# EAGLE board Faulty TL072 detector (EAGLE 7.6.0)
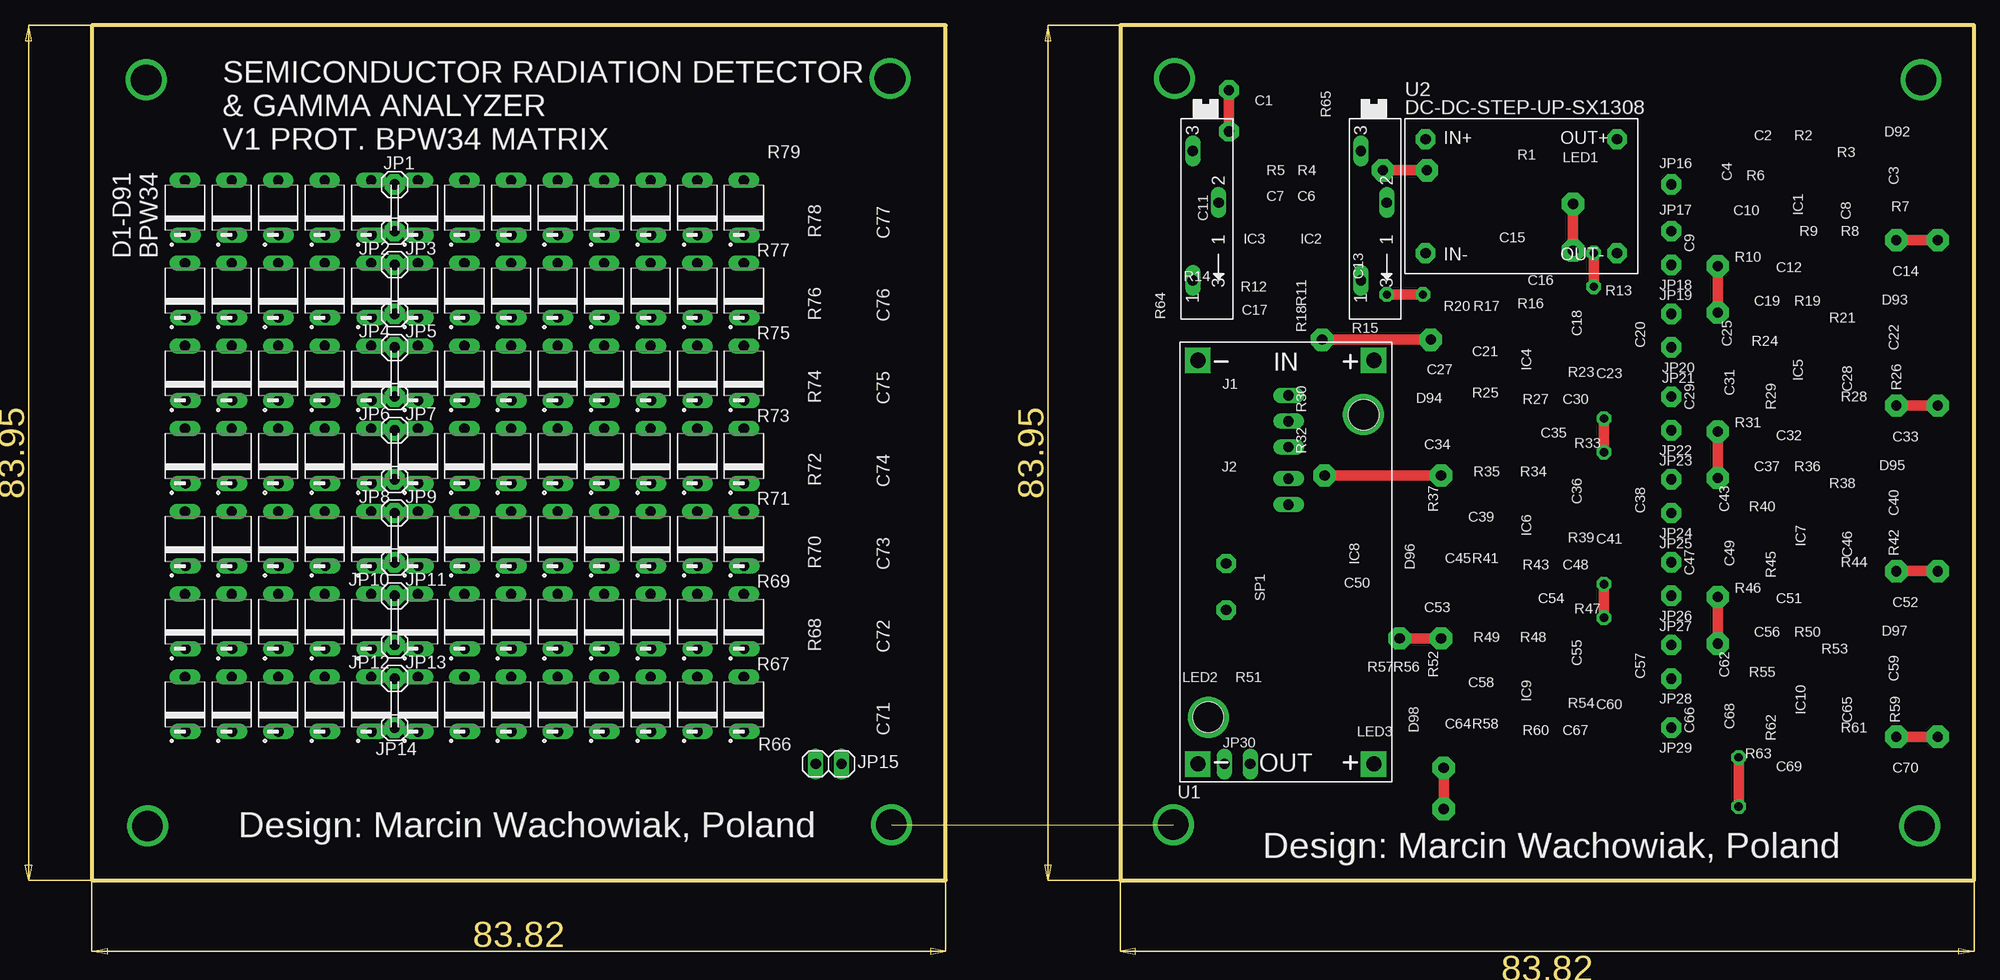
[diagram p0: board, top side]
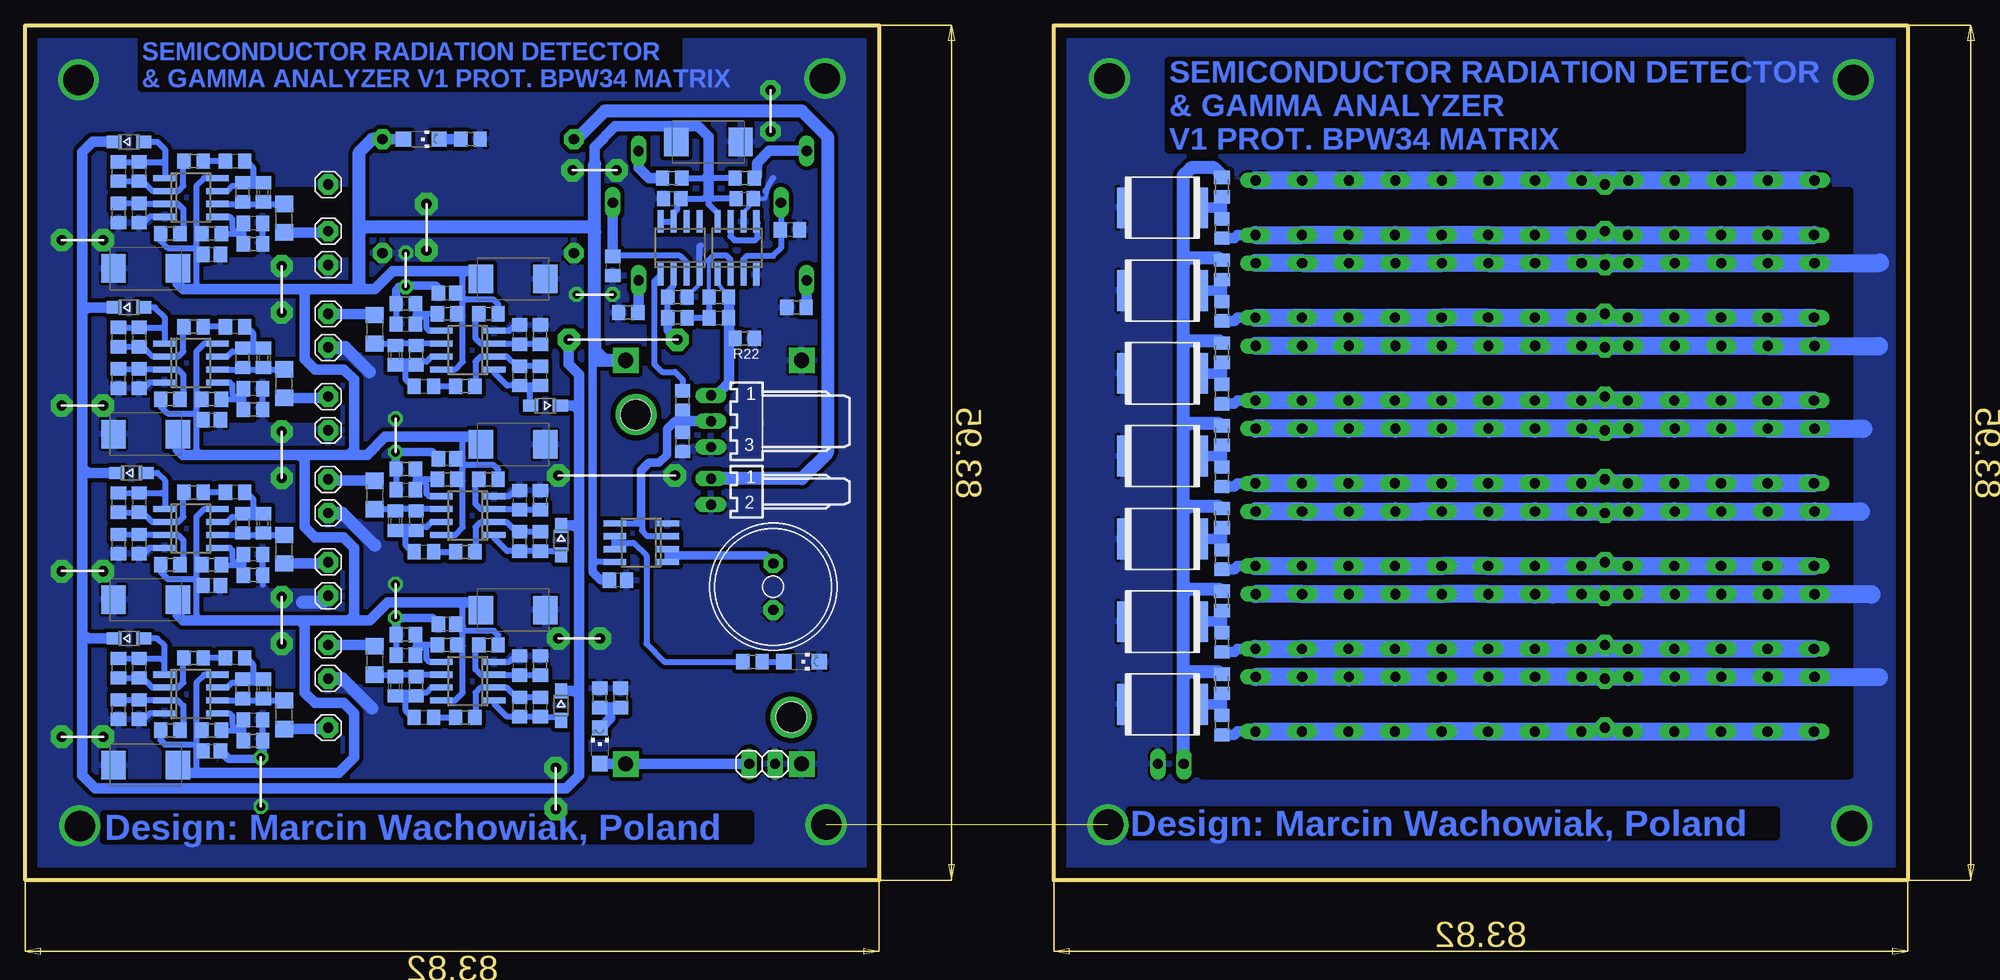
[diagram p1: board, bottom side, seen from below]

Size 191.31 x 91.23 mm. Coordinates in mm from the lower left corner, seen from the top.
Outline: 6.52,91.23 6.52,7.29 90.34,7.29 90.34,91.23 6.52,91.23
Outline: 191.31,91.23 107.49,91.23 107.49,7.29 191.31,7.29 191.31,91.23
Copper layers (1*16): Top 0.035mm / dielectric 1.5mm / Bottom 0.035mm
Design rules "default": minimum track width 10mil, minimum drill 24mil, track to track 8mil, track to pad 8mil, pad to pad 8mil, via to via 8mil, smd to smd 8mil, copper to edge 40mil, drill to drill 8mil, minimum pad ring 10mil, minimum via ring 8mil, stop-mask expansion 4mil, vias tented up to drill 0mil, thermal gap 10mil
bRestrict: area 159.6,68.9 to 166.9,75; area 160.8,36.4 to 167.2,40.2; area 160.8,20.6 to 167.2,24.4; area 160.8,19.3 to 167.2,20.6; area 160.8,52.6 to 167.2,56.7; area 155,59.5 to 162.9,64.6; area 155,43.2 to 162.9,48.3; area 155,27 to 162.9,32.1; area 12.2,17.6 to 72.4,75; area 72.4,22.7 to 75.7,75.7; area 72.4,17.6 to 75.7,22.7; area 167.2,18.7 to 172,20.6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

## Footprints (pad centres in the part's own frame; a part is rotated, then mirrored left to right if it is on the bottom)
SMC_D = smd 2.4 x 2.8: + -3.15,0; - 3.15,0
C0805 = smd 1.3 x 1.5: 1 -0.95,0; 2 0.95,0
C0603 = smd 1.1 x 1: 1 -0.85,0; 2 0.85,0
C0805' = smd 1.3 x 1.5: 1 -0.85,0; 2 0.85,0
C1206 = smd 1.6 x 1.8: 1 -1.4,0; 2 1.4,0
2824 = smd 1.2 x 4: 1 -3.85,0; 2 3.85,0
PHODET_BPW34 = drill 1 long: A 2.699,0.001; C -2.667,-0.033
SOD323-W = smd 1.5 x 1.2: A 1.45,0; C -1.45,0
SO08 = smd 0.6 x 2.2: 1 -1.905,-2.6; 2 -0.635,-2.6; 3 0.635,-2.6; 4 1.905,-2.6; 5 1.905,2.6; 6 0.635,2.6; 7 -0.635,2.6; 8 -1.905,2.6
7395-03 = drill 1.016 long: 1 2.54,0; 2 0,0; 3 -2.54,0
7395-02 = drill 1.016 long: 1 1.27,0; 2 -1.27,0
1X01 = drill 1.016 pad 2 octagon: 1 0,0
1X02 = drill 1.016 long: 1 -1.27,0; 2 1.27,0
CHIPLED_1206 = smd 1.5 x 1.5: A 0,-1.75; C 0,1.75
R0805 = smd 1.3 x 1.5: 1 -0.95,0; 2 0.95,0
SP19L = drill 1.016 long: A 5.715,-1.27; E -6.985,-1.27; S -1.905,1.27
M0805 = smd 1.3 x 1.6: 1 -0.95,0; 2 0.95,0
AL11P = drill 1.016 pad 1.905 octagon: + 2.286,0; - -2.286,0
DC-DC-STEP-DOWN-LM2596 = drill 1.5 pad 2.5 square: IN+ -19.812,8.636; IN- -19.812,-8.636; OUT+ 19.812,8.636; OUT- 19.812,-8.636 | hole 3: -14.478,7.62; 15.24,-7.62
DC-DC-STEP-UP-SX1308 = drill 1 pad 1.93 octagon: IN+ -9.398,5.588; IN- -9.398,-5.588; OUT+ 9.398,5.588; OUT- 9.398,-5.588

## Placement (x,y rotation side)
C1  100u/25V  [SMC_D]  124.25,79.8 0 bottom
C2  22n  [C0805]  170.73,77.9 180 bottom
C3  10p  [C0805]  182.16,76.88 270 bottom
C4  0,5pF  [C0603]  167.94,74.85 270 bottom
C5  0,5/1p  [C0805]  167.94,74.85 270 bottom
C6  100n  [C0805']  127.81,74.21 180 bottom
C7  100n  [C0805']  120.7,74.21 0 bottom
C8  100n  [C0805]  180.13,72.82 90 bottom
C9  100n/100V  [C1206]  165.91,72.31 90 bottom
C10  100n  [C0805]  168.96,71.8 180 bottom
C11  100n  [C0805]  116.25,71.17 180 bottom
C12  100n  [C0805']  173.02,68.75 0 bottom
C13  100n  [C0805]  133.65,67.61 270 bottom
C14  100u/25V  [SMC_D]  179.5,67.36 180 bottom
C15  100u/25V  [SMC_D]  143.43,66.34 0 bottom
C16  100n  [C0805']  149.91,64.94 180 bottom
C17  10p  [C0805]  123.24,62.53 0 bottom
C18  100n  [C0805]  153.97,61.89 0 bottom
C19  22n  [C0805]  170.73,61.64 180 bottom
C20  100n/100V  [C1206]  157.02,61.39 270 bottom
C21  100n  [C0805]  142.79,60.88 270 bottom
C22  10p  [C0805]  182.16,60.62 270 bottom
C23  0,5pF  [C0603]  154.99,58.85 90 bottom
C24  0,5/1p  [C0805]  154.99,58.85 90 bottom
C25  0,5/1p  [C0603]  167.94,58.59 270 bottom
C26  0,5/1p  [C0805]  167.94,58.59 270 bottom
C27  10p  [C0805]  140.76,56.81 90 bottom
C28  100n  [C0805]  180.13,56.56 90 bottom
C29  100n/100V  [C1206]  165.91,56.05 90 bottom
C30  22n  [C0805]  152.19,55.8 0 bottom
C31  100n  [C0805]  168.96,55.55 180 bottom
C32  100n  [C0805']  173.02,52.5 0 bottom
C33  100u/25V  [SMC_D]  179.5,51.1 180 bottom
C34  100u/25V  [SMC_D]  143.43,50.08 0 bottom
C35  100n  [C0805']  149.91,48.69 180 bottom
C36  100n  [C0805]  153.97,45.64 0 bottom
C37  22n  [C0805]  170.73,45.39 180 bottom
C38  100n/100V  [C1206]  157.02,45.13 270 bottom
C39  100n  [C0805]  142.79,44.62 270 bottom
C40  10p  [C0805]  182.16,44.37 270 bottom
C41  0,5pF  [C0603]  154.99,42.59 90 bottom
C42  0,5/1p  [C0805]  154.99,42.59 90 bottom
C43  0,5pF  [C0603]  167.94,42.34 270 bottom
C44  0,5/1p  [C0805]  167.94,42.34 270 bottom
C45  10p  [C0805]  140.76,40.56 90 bottom
C46  100n  [C0805]  180.13,40.31 90 bottom
C47  100n/100V  [C1206]  165.91,39.8 90 bottom
C48  22n  [C0805]  152.19,39.54 0 bottom
C49  100n  [C0805]  168.96,39.29 180 bottom
C50  100n  [C0805']  133.14,36.75 180 bottom
C51  100n  [C0805']  173.02,36.24 0 bottom
C52  100u/25V  [SMC_D]  179.5,34.84 180 bottom
C53  100u/25V  [SMC_D]  143.43,33.83 0 bottom
C54  100n  [C0805']  149.91,32.43 180 bottom
C55  100n  [C0805]  153.97,29.38 0 bottom
C56  22n  [C0805]  170.73,29.13 180 bottom
C57  100n/100V  [C1206]  157.02,28.88 270 bottom
C58  100n  [C0805]  142.79,28.37 270 bottom
C59  10p  [C0805]  182.16,28.11 270 bottom
C60  0,5pF  [C0603]  154.99,26.34 90 bottom
C61  0,5/1p  [C0805]  154.99,26.34 90 bottom
C62  0,5pF  [C0603]  167.94,26.08 270 bottom
C63  0,5/1p  [C0805]  167.94,26.08 270 bottom
C64  10p  [C0805]  140.76,24.3 90 bottom
C65  100n  [C0805]  180.13,24.05 90 bottom
C66  100n/100V  [C1206]  165.91,23.54 90 bottom
C67  22n  [C0805]  152.19,23.29 0 bottom
C68  100n  [C0805]  168.96,23.03 180 bottom
C69  100n  [C0805']  173.02,19.98 0 bottom
C70  100u/25V  [SMC_D]  179.5,18.59 180 bottom
C71  2,2uF/100V  [2824]  79.67,24.56 180 bottom
C72  2,2uF/100V  [2824]  79.67,32.69 180 bottom
C73  2,2uF/100V  [2824]  79.67,40.81 180 bottom
C74  2,2uF/100V  [2824]  79.67,48.94 180 bottom
C75  2,2uF/100V  [2824]  79.67,57.07 180 bottom
C76  2,2uF/100V  [2824]  79.67,65.2 180 bottom
C77  2,2uF/100V  [2824]  79.67,73.33 180 bottom
D1  BPW34  [PHODET_BPW34]  15.67,73.33 90 top
D2  BPW34  [PHODET_BPW34]  20.24,73.33 90 top
D3  BPW34  [PHODET_BPW34]  24.81,73.33 90 top
D4  BPW34  [PHODET_BPW34]  29.38,73.33 90 top
D5  BPW34  [PHODET_BPW34]  33.95,73.33 90 top
D6  BPW34  [PHODET_BPW34]  38.53,73.33 90 top
D7  BPW34  [PHODET_BPW34]  43.1,73.33 90 top
D8  BPW34  [PHODET_BPW34]  47.67,73.33 90 top
D9  BPW34  [PHODET_BPW34]  52.24,73.33 90 top
D10  BPW34  [PHODET_BPW34]  56.81,73.33 90 top
D11  BPW34  [PHODET_BPW34]  61.39,73.33 90 top
D12  BPW34  [PHODET_BPW34]  65.96,73.33 90 top
D13  BPW34  [PHODET_BPW34]  70.53,73.33 90 top
D14  BPW34  [PHODET_BPW34]  15.67,65.2 90 top
D15  BPW34  [PHODET_BPW34]  20.24,65.2 90 top
D16  BPW34  [PHODET_BPW34]  24.81,65.2 90 top
D17  BPW34  [PHODET_BPW34]  29.38,65.2 90 top
D18  BPW34  [PHODET_BPW34]  33.95,65.2 90 top
D19  BPW34  [PHODET_BPW34]  38.53,65.2 90 top
D20  BPW34  [PHODET_BPW34]  43.1,65.2 90 top
D21  BPW34  [PHODET_BPW34]  47.67,65.2 90 top
D22  BPW34  [PHODET_BPW34]  52.24,65.2 90 top
D23  BPW34  [PHODET_BPW34]  56.81,65.2 90 top
D24  BPW34  [PHODET_BPW34]  61.39,65.2 90 top
D25  BPW34  [PHODET_BPW34]  65.96,65.2 90 top
D26  BPW34  [PHODET_BPW34]  70.53,65.2 90 top
D27  BPW34  [PHODET_BPW34]  15.67,57.07 90 top
D28  BPW34  [PHODET_BPW34]  20.24,57.07 90 top
D29  BPW34  [PHODET_BPW34]  24.81,57.07 90 top
D30  BPW34  [PHODET_BPW34]  29.38,57.07 90 top
D31  BPW34  [PHODET_BPW34]  33.95,57.07 90 top
D32  BPW34  [PHODET_BPW34]  38.53,57.07 90 top
D33  BPW34  [PHODET_BPW34]  43.1,57.07 90 top
D34  BPW34  [PHODET_BPW34]  47.67,57.07 90 top
D35  BPW34  [PHODET_BPW34]  52.24,57.07 90 top
D36  BPW34  [PHODET_BPW34]  56.81,57.07 90 top
D37  BPW34  [PHODET_BPW34]  61.39,57.07 90 top
D38  BPW34  [PHODET_BPW34]  65.96,57.07 90 top
D39  BPW34  [PHODET_BPW34]  70.53,57.07 90 top
D40  BPW34  [PHODET_BPW34]  15.67,48.94 90 top
D41  BPW34  [PHODET_BPW34]  20.24,48.94 90 top
D42  BPW34  [PHODET_BPW34]  24.81,48.94 90 top
D43  BPW34  [PHODET_BPW34]  29.38,48.94 90 top
D44  BPW34  [PHODET_BPW34]  33.95,48.94 90 top
D45  BPW34  [PHODET_BPW34]  38.53,48.94 90 top
D46  BPW34  [PHODET_BPW34]  43.1,48.94 90 top
D47  BPW34  [PHODET_BPW34]  47.67,48.94 90 top
D48  BPW34  [PHODET_BPW34]  52.24,48.94 90 top
D49  BPW34  [PHODET_BPW34]  56.81,48.94 90 top
D50  BPW34  [PHODET_BPW34]  61.39,48.94 90 top
D51  BPW34  [PHODET_BPW34]  65.96,48.94 90 top
D52  BPW34  [PHODET_BPW34]  70.53,48.94 90 top
D53  BPW34  [PHODET_BPW34]  15.67,40.81 90 top
D54  BPW34  [PHODET_BPW34]  20.24,40.81 90 top
D55  BPW34  [PHODET_BPW34]  24.81,40.81 90 top
D56  BPW34  [PHODET_BPW34]  29.38,40.81 90 top
D57  BPW34  [PHODET_BPW34]  33.95,40.81 90 top
D58  BPW34  [PHODET_BPW34]  38.53,40.81 90 top
D59  BPW34  [PHODET_BPW34]  43.1,40.81 90 top
D60  BPW34  [PHODET_BPW34]  47.67,40.81 90 top
D61  BPW34  [PHODET_BPW34]  52.24,40.81 90 top
D62  BPW34  [PHODET_BPW34]  56.81,40.81 90 top
D63  BPW34  [PHODET_BPW34]  61.39,40.81 90 top
D64  BPW34  [PHODET_BPW34]  65.96,40.81 90 top
D65  BPW34  [PHODET_BPW34]  70.53,40.81 90 top
D66  BPW34  [PHODET_BPW34]  15.67,32.69 90 top
D67  BPW34  [PHODET_BPW34]  20.24,32.69 90 top
D68  BPW34  [PHODET_BPW34]  24.81,32.69 90 top
D69  BPW34  [PHODET_BPW34]  29.38,32.69 90 top
D70  BPW34  [PHODET_BPW34]  33.95,32.69 90 top
D71  BPW34  [PHODET_BPW34]  38.53,32.69 90 top
D72  BPW34  [PHODET_BPW34]  43.1,32.69 90 top
D73  BPW34  [PHODET_BPW34]  47.67,32.69 90 top
D74  BPW34  [PHODET_BPW34]  52.24,32.69 90 top
D75  BPW34  [PHODET_BPW34]  56.81,32.69 90 top
D76  BPW34  [PHODET_BPW34]  61.39,32.69 90 top
D77  BPW34  [PHODET_BPW34]  65.96,32.69 90 top
D78  BPW34  [PHODET_BPW34]  70.53,32.69 90 top
D79  BPW34  [PHODET_BPW34]  15.67,24.56 90 top
D80  BPW34  [PHODET_BPW34]  20.24,24.56 90 top
D81  BPW34  [PHODET_BPW34]  24.81,24.56 90 top
D82  BPW34  [PHODET_BPW34]  29.38,24.56 90 top
D83  BPW34  [PHODET_BPW34]  33.95,24.56 90 top
D84  BPW34  [PHODET_BPW34]  38.53,24.56 90 top
D85  BPW34  [PHODET_BPW34]  43.1,24.56 90 top
D86  BPW34  [PHODET_BPW34]  47.67,24.56 90 top
D87  BPW34  [PHODET_BPW34]  52.24,24.56 90 top
D88  BPW34  [PHODET_BPW34]  56.81,24.56 90 top
D89  BPW34  [PHODET_BPW34]  61.39,24.56 90 top
D90  BPW34  [PHODET_BPW34]  65.96,24.56 90 top
D91  BPW34  [PHODET_BPW34]  70.53,24.56 90 top
D92  1N4448  [SOD323-W]  181.15,79.8 0 bottom
D93  1N4448  [SOD323-W]  181.15,63.55 0 bottom
D94  1N4448  [SOD323-W]  140.25,53.89 180 bottom
D95  1N4448  [SOD323-W]  180.89,47.29 0 bottom
D96  1N4448  [SOD323-W]  138.73,40.69 270 bottom
D97  1N4448  [SOD323-W]  181.15,31.03 0 bottom
D98  1N4448  [SOD323-W]  138.73,24.43 270 bottom
IC1  TL072  [SO08]  175.05,74.34 270 bottom
IC2  LM311  [SO08]  127.05,69.39 0 bottom
IC3  LM358  [SO08]  121.46,69.39 0 bottom
IC4  TL072  [SO08]  147.87,59.36 90 bottom
IC5  TL072  [SO08]  175.05,58.09 270 bottom
IC6  TL072  [SO08]  147.87,43.1 90 bottom
IC7  TL072  [SO08]  175.05,41.83 270 bottom
IC8  LM358  [SO08]  130.86,40.43 90 bottom
IC9  TL072  [SO08]  147.87,26.84 90 bottom
IC10  TL072  [SO08]  175.05,25.57 270 bottom
J1  3pin  [7395-03]  124,52.37 90 bottom
J2  2pin  [7395-02]  124,45.45 90 bottom
JP1  [1X01]  36.24,75.61 0 top
JP2  [1X01]  36.24,71.04 0 top
JP3  [1X01]  36.24,67.74 0 top
JP4  [1X01]  36.24,62.91 0 top
JP5  [1X01]  36.24,59.61 0 top
JP6  [1X01]  36.24,54.78 0 top
JP7  [1X01]  36.24,51.48 0 top
JP8  [1X01]  36.24,46.66 0 top
JP9  [1X01]  36.24,43.35 0 top
JP10  [1X01]  36.24,38.53 0 top
JP11  [1X01]  36.24,35.23 0 top
JP12  [1X01]  36.24,30.4 0 top
JP13  [1X01]  36.24,27.1 0 top
JP14  [1X01]  36.24,22.27 0 top
JP15  GP  [1X02]  78.85,18.72 180 top
JP16  [1X01]  161.59,75.61 0 bottom
JP17  [1X01]  161.59,71.04 0 bottom
JP18  [1X01]  161.59,67.74 0 bottom
JP19  [1X01]  161.59,62.91 0 bottom
JP20  [1X01]  161.59,59.61 0 bottom
JP21  [1X01]  161.59,54.78 0 bottom
JP22  [1X01]  161.59,51.48 0 bottom
JP23  [1X01]  161.59,46.66 0 bottom
JP24  [1X01]  161.59,43.35 0 bottom
JP25  [1X01]  161.59,38.53 0 bottom
JP26  [1X01]  161.59,35.23 0 bottom
JP27  [1X01]  161.59,30.4 0 bottom
JP28  [1X01]  161.59,27.1 0 bottom
JP29  [1X01]  161.59,22.27 0 bottom
JP30  [1X02]  118.98,18.72 0 bottom
LED1  GREEN  [CHIPLED_1206]  152.45,80.06 270 bottom
LED2  RED  [CHIPLED_1206]  115.11,28.75 270 bottom
LED3  GREEN  [CHIPLED_1206]  134.92,20.49 0 bottom
R1  3k  [R0805]  147.62,80.06 0 bottom
R2  1k  [R0805]  174.8,77.9 0 bottom
R3  100k  [R0805]  180.13,76.88 270 bottom
R4  1k  [R0805]  127.81,76.25 180 bottom
R5  1k  [R0805]  120.7,76.25 180 bottom
R6  10M  [R0805]  169.97,74.85 270 bottom
R7  10k  [R0805]  182.16,72.82 270 bottom
R8  10k  [R0805]  177.08,70.78 0 bottom
R9  10k  [R0805]  173.02,70.78 0 bottom
R10  10k  [R0805]  168.96,69.77 0 bottom
R11  10k  [R0805]  127.3,64.56 0 bottom
R12  ***  [R0805]  123.24,64.56 0 bottom
R13  10k  [R0805]  153.97,63.93 180 bottom
R14  1k  [R0805]  115.62,63.55 0 bottom
R15  1k  [R0805]  132.13,63.04 180 bottom
R16  10k  [R0805]  149.91,62.91 180 bottom
R17  10k  [R0805]  145.84,62.91 180 bottom
R18  10k  [R0805]  127.3,62.53 0 bottom
R19  1k  [R0805]  174.8,61.64 0 bottom
R20  10k  [R0805]  140.76,60.88 90 bottom
R21  100k  [R0805]  180.13,60.62 270 bottom
R22  10k  [R0805]  120.7,60.5 180 bottom
R23  10M  [R0805]  152.95,58.85 90 bottom
R24  10M  [R0805]  169.97,58.59 270 bottom
R25  100k  [R0805]  142.79,56.81 90 bottom
R26  10k  [R0805]  182.16,56.56 270 bottom
R27  1k  [R0805]  148.13,55.8 180 bottom
R28  10k  [R0805]  177.08,54.53 0 bottom
R29  10k  [R0805]  173.02,54.53 0 bottom
R30  1200  [R0805]  126.79,54.4 270 bottom
R31  10k  [R0805]  168.96,53.51 0 bottom
R32  560  [R0805]  126.79,50.34 270 bottom
R33  10k  [R0805]  153.97,47.67 180 bottom
R34  10k  [R0805]  149.91,46.66 180 bottom
R35  10k  [R0805]  145.84,46.66 180 bottom
R36  1k  [R0805]  174.8,45.39 0 bottom
R37  10k  [R0805]  140.76,44.62 90 bottom
R38  100k  [R0805]  180.13,44.37 270 bottom
R39  10M  [R0805]  152.95,42.59 90 bottom
R40  10M  [R0805]  169.97,42.34 270 bottom
R41  100k  [R0805]  142.79,40.56 90 bottom
R42  10k  [R0805]  182.16,40.31 270 bottom
R43  1k  [R0805]  148.13,39.54 180 bottom
R44  10k  [R0805]  177.08,38.27 0 bottom
R45  10k  [R0805]  173.02,38.27 0 bottom
R46  10k  [R0805]  168.96,37.26 0 bottom
R47  10k  [R0805]  153.97,31.41 180 bottom
R48  10k  [R0805]  149.91,30.4 180 bottom
R49  10k  [R0805]  145.84,30.4 180 bottom
R50  1k  [R0805]  174.8,29.13 0 bottom
R51  470  [R0805]  119.93,28.75 180 bottom
R52  10k  [R0805]  140.76,28.37 90 bottom
R53  100k  [R0805]  180.13,28.11 270 bottom
R54  10M  [R0805]  152.95,26.34 90 bottom
R55  10M  [R0805]  169.97,26.08 270 bottom
R56  20k  [R0805]  134.92,25.19 90 bottom
R57  20k  [R0805]  132.89,25.19 90 bottom
R58  100k  [R0805]  142.79,24.3 90 bottom
R59  10k  [R0805]  182.16,24.05 270 bottom
R60  1k  [R0805]  148.13,23.29 180 bottom
R61  10k  [R0805]  177.08,22.02 0 bottom
R62  10k  [R0805]  173.02,22.02 0 bottom
R63  10k  [R0805]  168.96,21 0 bottom
R64  100-330 prec  [SP19L]  115.87,71.93 270 top
R65  100-330 prec  [SP19L]  132.38,71.93 270 top
R66  100M  [R0805]  73.83,22.52 270 bottom
R67  1M  [M0805]  73.83,26.59 270 bottom
R68  100M  [R0805]  73.83,30.65 270 bottom
R69  1M  [M0805]  73.83,34.72 270 bottom
R70  100M  [R0805]  73.83,38.78 270 bottom
R71  1M  [M0805]  73.83,42.84 270 bottom
R72  100M  [R0805]  73.83,46.91 270 bottom
R73  1M  [M0805]  73.83,50.97 270 bottom
R74  100M  [R0805]  73.83,55.04 270 bottom
R75  1M  [M0805]  73.83,59.1 270 bottom
R76  100M  [R0805]  73.83,63.17 270 bottom
R77  1M  [M0805]  73.83,67.23 270 bottom
R78  100M  [R0805]  73.83,71.29 270 bottom
R79  1M  [M0805]  73.83,75.36 270 bottom
SP1  BUZ  [AL11P]  117.9,36.11 90 bottom
U1  DC-DC-STEP-UP-LM2596  [DC-DC-STEP-DOWN-LM2596]  123.74,38.53 270 top
U2  DC-DC-STEP-UP-SX1308  [DC-DC-STEP-UP-SX1308]  146.86,74.47 0 top

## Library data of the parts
C1-C5 C8-C11 C13-C15 C17-C31 C33 C34 C36-C49 C52 C53 C55-C68 C70 R1-R63 R66-R79 = rcl
C6 C7 C12 C16 C32 C35 C50 C51 C54 C69 = resistor
C71-C77 = capacitor-wima
D1-D91 = BPW34; AVAILABILITY: Good; DESCRIPTION: 950 nm 100 ns %C2%B1 65%C2%B0 Wide Angle Half Sensitivity TO-5 Silicon PIN Photodiode; MF: Vishay; MP: BPW34; PACKAGE: SMD-2 Vishay; PRICE: 0.62 USD
D92-D98 = diode
IC1-IC10 = linear
J1 = con-molex; OC_FARNELL: unknown; OC_NEWARK: unknown
J2 = con-molex; OC_FARNELL: 9731601; OC_NEWARK: unknown
JP1-JP30 = pinhead
LED1-LED3 = led
R64 R65 = pot
SP1 = buzzer; OC_FARNELL: unknown; OC_NEWARK: unknown
U1 U2 = diy-modules

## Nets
+18V: C1.+ C6.1 C7.1 C12.1 C14.+ C15.+ C16.1 C32.1 C33.+ C34.+ C35.1 C50.2 C51.1 C52.+ C53.+ C54.1 C69.1 C70.+ IC1.8 IC2.7 IC2.8 IC3.8 IC4.8 IC5.8 IC6.8 IC7.8 IC8.8 IC9.8 IC10.8 LED1.A R4.1 R5.2 R8.1 R9.1 R16.1 R17.1 R28.1 R29.1 R34.1 R35.1 R44.1 R45.1 R48.1 R49.1 R61.1 R62.1 U1.IN+ U2.OUT+
+24V: JP30.1 LED3.A U1.OUT+
+60: JP15.2 R67.1 R69.1 R71.1 R73.1 R75.1 R77.1 R79.1
A-OUT: C17.2 IC3.1 J1.1 R12.2 R22.2
D-OUT+5V: IC8.3 IC8.5 J1.2 R30.2 R32.1
GND: C1.- C6.2 C7.2 C8.1 C10.1 C11.1 C12.2 C13.2 C14.- C15.- C16.2 C18.1 C21.1 C28.1 C31.1 C32.2 C33.- C34.- C35.2 C36.1 C39.1 C46.1 C49.1 C50.1 C51.2 C52.- C53.- C54.2 C55.1 C58.1 C65.1 C68.1 C69.2 C70.- C71.2 C72.2 C73.2 C74.2 C75.2 C76.2 C77.2 D1.A D2.A D3.A D4.A D5.A D6.A D7.A D8.A D9.A D10.A D11.A D12.A D13.A D14.A D15.A D16.A D17.A D18.A D19.A D20.A D21.A D22.A D23.A D24.A D25.A D26.A D27.A D28.A D29.A D30.A D31.A D32.A D33.A D34.A D35.A D36.A D37.A D38.A D39.A D40.A D41.A D42.A D43.A D44.A D45.A D46.A D47.A D48.A D49.A D50.A D51.A D52.A D53.A D54.A D55.A D56.A D57.A D58.A D59.A D60.A D61.A D62.A D63.A D64.A D65.A D66.A D67.A D68.A D69.A D70.A D71.A D72.A D73.A D74.A D75.A D76.A D77.A D78.A D79.A D80.A D81.A D82.A D83.A D84.A D85.A D86.A D87.A D88.A D89.A D90.A D91.A IC1.4 IC2.4 IC3.4 IC3.6 IC4.4 IC5.4 IC6.4 IC7.4 IC8.4 IC9.4 IC10.4 J1.3 J2.2 JP1.1 JP3.1 JP5.1 JP7.1 JP9.1 JP11.1 JP13.1 JP15.1 JP16.1 JP18.1 JP20.1 JP22.1 JP24.1 JP26.1 JP28.1 JP30.2 LED2.C R1.2 R7.2 R10.2 R11.2 R13.2 R14.1 R15.2 R20.2 R22.1 R26.2 R31.2 R32.2 R33.2 R37.2 R42.2 R46.2 R47.2 R52.2 R56.2 R57.2 R59.2 R63.2 SP1.- U1.IN- U1.OUT- U2.IN- U2.OUT-
N$1: C10.2 IC1.5 R9.2 R10.1
N$3: C2.1 C4.1 C5.1 IC1.7 R6.1
N$4: J2.1 U2.IN+
N$5: C77.1 R78.1 R79.2
N$6: C8.2 IC1.3 R7.1 R8.2
N$7: C2.2 R2.2
N$8: C4.2 C5.2 C9.2 IC1.6 R6.2
N$9: C3.2 IC1.2 R2.1 R3.2
N$10: C3.1 D92.A IC1.1 R3.1
N$12: D92.C D93.C D94.C D95.C D96.C D97.C D98.C IC2.2 R11.1 R18.1
N$13: C76.1 R76.1 R77.2
N$14: C75.1 R74.1 R75.2
N$15: C74.1 R72.1 R73.2
N$16: C73.1 R70.1 R71.2
N$17: C72.1 R68.1 R69.2
N$18: C71.1 R66.1 R67.2
N$23: IC2.1 R30.1
N$24: C17.1 IC3.2 R12.1 R18.2
N$25: C13.1 IC2.3 R65.S
N$26: R4.2 R65.E
N$27: R15.1 R65.A
N$28: C25.2 C26.2 C29.2 IC5.6 R24.2
N$29: R5.1 R64.E
N$30: R14.2 R64.A
N$31: C11.2 IC3.3 R64.S
N$32: LED1.C R1.1
N$33: C31.2 IC5.5 R29.2 R31.1
N$34: LED3.C R56.1 R57.1
N$35: C19.1 C25.1 C26.1 IC5.7 R24.1
N$36: C19.2 R19.2
N$37: C22.2 IC5.2 R19.1 R21.2
N$38: C22.1 D93.A IC5.1 R21.1
N$39: C28.2 IC5.3 R26.1 R28.2
N$40: C38.2 C41.2 C42.2 IC6.6 R39.2
N$41: C36.2 IC6.5 R33.1 R34.2
N$42: C43.2 C44.2 C47.2 IC7.6 R40.2
N$43: C49.2 IC7.5 R45.2 R46.1
N$44: C37.1 C43.1 C44.1 IC7.7 R40.1
N$45: C37.2 R36.2
N$46: C40.2 IC7.2 R36.1 R38.2
N$47: C40.1 D95.A IC7.1 R38.1
N$48: C46.2 IC7.3 R42.1 R44.2
N$49: C41.1 C42.1 C48.1 IC6.7 R39.1
N$50: C48.2 R43.2
N$51: C62.2 C63.2 C66.2 IC10.6 R55.2
N$52: C68.2 IC10.5 R62.2 R63.1
N$53: C56.1 C62.1 C63.1 IC10.7 R55.1
N$54: C56.2 R50.2
N$55: C59.2 IC10.2 R50.1 R53.2
N$56: C59.1 D97.A IC10.1 R53.1
N$57: C65.2 IC10.3 R59.1 R61.2
N$58: C45.2 IC6.2 R41.2 R43.1
N$59: C45.1 D96.A IC6.1 R41.1
N$60: C20.2 C23.2 C24.2 IC4.6 R23.2
N$61: C18.2 IC4.5 R13.1 R16.2
N$62: C23.1 C24.1 C30.1 IC4.7 R23.1
N$63: C30.2 R27.2
N$64: C27.2 IC4.2 R25.2 R27.1
N$65: C27.1 D94.A IC4.1 R25.1
N$66: C21.2 IC4.3 R17.2 R20.1
N$67: C39.2 IC6.3 R35.2 R37.1
N$69: C57.2 C60.2 C61.2 IC9.6 R54.2
N$70: C55.2 IC9.5 R47.1 R48.2
N$71: C60.1 C61.1 C67.1 IC9.7 R54.1
N$72: C67.2 R60.2
N$73: C64.2 IC9.2 R58.2 R60.1
N$74: C64.1 D98.A IC9.1 R58.1
N$75: C58.2 IC9.3 R49.2 R52.1
N$78: IC8.1 IC8.2 SP1.+
N$79: IC8.6 IC8.7 R51.2
OUT1: D27.C D28.C D29.C D30.C D31.C D32.C D33.C D34.C D35.C D36.C D37.C D38.C D39.C JP6.1 R74.2
OUT3: D79.C D80.C D81.C D82.C D83.C D84.C D85.C D86.C D87.C D88.C D89.C D90.C D91.C JP14.1 R66.2
OUT4: D1.C D2.C D3.C D4.C D5.C D6.C D7.C D8.C D9.C D10.C D11.C D12.C D13.C JP2.1 R78.2
OUT5: D14.C D15.C D16.C D17.C D18.C D19.C D20.C D21.C D22.C D23.C D24.C D25.C D26.C JP4.1 R76.2
OUT9: D40.C D41.C D42.C D43.C D44.C D45.C D46.C D47.C D48.C D49.C D50.C D51.C D52.C JP8.1 R72.2
OUT10: C9.1 JP17.1
OUT12: C20.1 JP19.1
OUT13: C66.1 JP29.1
OUT14: C29.1 JP21.1
OUT15: C38.1 JP23.1
OUT16: C47.1 JP25.1
OUT17: C57.1 JP27.1
OUT21: D53.C D54.C D55.C D56.C D57.C D58.C D59.C D60.C D61.C D62.C D63.C D64.C D65.C JP10.1 R70.2
OUT22: D66.C D67.C D68.C D69.C D70.C D71.C D72.C D73.C D74.C D75.C D76.C D77.C D78.C JP12.1 R68.2
S$1: IC3.5 IC3.7
S$2: LED2.A R51.1

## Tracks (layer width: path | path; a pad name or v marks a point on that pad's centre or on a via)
+18V
  Bottom 0.61: IC4.8 149.14,57.45 148.38,58.21 148.38,62.78 | R16.1 148.51,62.91 148.38,62.78 | IC10.8 173.78,27.48 174.54,26.72 174.54,22.14 | C69.1 174,19.86 174.54,19.86 | R62.1 174.42,22.02 174.54,22.14 | IC7.8 173.78,43.73 174.54,42.97 174.54,38.4 | R45.1 174.42,38.27 174.54,38.4 | IC5.8 173.78,59.99 174.54,59.23 174.54,54.66 | C32.1 174,52.37 174.29,52.37 174.54,52.62 | R29.1 174.42,54.53 174.54,54.66 | IC1.8 173.78,76.25 174.54,75.48 174.54,70.91 | 174,68.63 C12.1 174.25,69.13 174.54,69.13 | R9.1 174.42,70.78 174.54,70.91 | 126.86,74.57 C6.1 | 126.86,79 C1.+ | IC6.8 149.14,41.19 148.38,41.96 148.38,46.53 | 148.38,46.53 148.38,48.05 | R34.1 148.51,46.66 148.38,46.53 | IC9.8 149.14,24.94 148.38,25.7 148.38,30.27 | 148.38,30.27 148.38,31.8 | R48.1 148.51,30.4 148.38,30.27 | 148.38,62.78 148.38,64.31 | 148.38,64.31 148.38,64.56 | 148.38,64.56 148.38,65.07 | C16.1 148.51,64.94 148.38,65.07 | 174.54,70.91 174.54,69.13 | 174.54,69.13 174.54,65.83 | 174.54,65.83 174.54,65.32 | R8.1 178.03,70.08 177.34,69.39 174.8,69.39 174.54,69.13 | R17.1 144.89,63.87 145.33,64.31 148.13,64.31 | 148.13,64.31 148.38,64.31 | 148.13,64.31 148.38,64.56 | 148.38,48.05 148.38,48.31 | 148.38,48.31 148.38,48.81 | 148.38,48.81 148.38,50.34 148.89,50.85 | 174.54,54.66 174.54,52.88 | 174.54,52.88 174.54,52.62 | 174.54,52.62 174.54,49.58 | R28.1 178.03,53.83 177.34,53.13 174.8,53.13 174.54,52.88 | R35.1 144.89,47.61 145.33,48.05 148.13,48.05 | 148.13,48.05 148.38,48.05 | 148.13,48.05 148.38,48.31 | C35.1 148.51,48.69 148.38,48.81 | 148.38,31.8 148.38,32.05 | 174.54,38.4 174.54,36.62 | 174.54,36.62 174.54,36.37 | 174.54,36.37 174.54,33.32 | 174.54,33.32 174.54,32.81
  Bottom 0.61: R44.1 178.03,37.57 177.34,36.88 174.8,36.88 174.54,36.62 | R49.1 144.89,31.35 145.33,31.8 148.13,31.8 | 148.13,31.8 148.38,31.8 | 148.13,31.8 148.38,32.05 | C51.1 174.42,36.24 174.54,36.37 | 148.38,32.05 148.38,32.3 | C54.1 148.51,32.43 148.38,32.3 | 148.38,32.3 148.38,34.08 148.89,34.59 | 174.54,33.32 174.29,33.07 174.29,32.81 | 174.54,49.07 174.54,49.58 | 174.54,49.58 173.78,49.07 | 174.54,65.83 174.04,65.32 | 148.38,65.07 148.38,66.59 148.89,67.1 | 174.54,22.14 174.54,20.37 | 174.54,20.37 174.54,19.86 | 174.54,19.86 174.54,18.33 174.04,17.83 | 177.08,18.08 176.85,18.08 C70.+ | R61.1 178.03,21.06 177.59,20.62 174.8,20.62 174.54,20.37 | IC2.8 IC2.7 127.68,72.82 127.3,73.2 127.3,73.87 C6.1 | R5.2 123.74,76.25 124.25,76.75 124.76,76.25 R4.1 | C6.1 124.76,74.21 | 124.76,74.21 124.51,74.47 | IC3.8 123.36,72.82 124.25,73.71 124.25,74.47 | 124.51,74.21 124.51,74.47 | 124.51,74.47 124.25,74.72 123.74,74.21 | C7.1 124.76,74.21 | 135.62,59.86 135.43,60.24 | IC8.8 135.24,38.53 135.62,38.91
  Bottom 0.813: 156.51,80.31 U2.OUT+ | 135.62,59.86 135.62,38.91 135.62,37.57 134.79,36.75 C50.2
  Bottom 1.016: C14.+ 176.35,65.86 175.81,65.32 174.54,65.32 174.04,65.32 164.38,65.32 | C33.+ 176.35,49.6 175.81,49.07 174.54,49.07 173.78,49.07 163.62,49.07 | C52.+ 176.35,33.34 175.81,32.81 174.54,32.81 174.29,32.81 164.38,32.81 | 164.38,32.81 159.56,32.81 | 159.56,32.81 159.3,32.81 | 159.56,49.07 159.05,49.58 159.05,56.43 160.07,57.45 162.86,57.45 163.88,58.47 163.88,65.07 164.38,65.32 | 159.43,32.94 159.05,33.32 159.05,39.92 160.07,40.94 162.86,40.94 163.88,41.96 163.88,48.56 164,48.69 | 159.43,32.94 159.56,32.81 | 164,48.69 164.38,49.07 | 159.56,49.07 163.62,49.07 | 163.62,49.07 164,48.69 | 159.3,32.81 159.43,32.94 | 176.09,18.33 C70.+ | 164.38,32.81 163.88,32.3 163.88,25.7 162.86,24.68 160.07,24.68 159.05,23.67 159.05,19.35 160.57,17.83 174.04,17.83 176.07,17.83 | 164.38,65.32 159.05,65.32 | 159.05,65.32 158.54,65.32 | 158.54,65.32 157.02,65.32 155.24,67.1 148.89,67.1 147.34,67.1 C15.+ | C1.+ 127.05,80.16 127.05,81.07 127.3,81.33 | 158.54,66.34 158.54,65.83 | 158.54,65.83 158.54,65.32 | 158.54,65.83 159.05,65.32 | LED1.A U2.OUT+ | 124.25,74.47 124.25,74.72 124.25,76.75 124.25,80.31 125.27,81.33 127.3,81.33 | 159.3,32.81 157.53,32.81 155.75,34.59 148.89,34.59 147.34,34.59 C53.+ | 159.56,49.07 157.78,49.07 156,50.85 148.89,50.85 147.34,50.85 C34.+ | 127.3,81.33 133.4,81.33 135.43,79.29 135.43,77.14
  Bottom 1.27: U2.OUT+ 157.27,80.06 158.54,78.79 158.54,70.91 | 158.54,65.83 158.54,70.91 | U1.IN+ 134.41,58.34 | 134.41,58.34 135.05,58.34 | 135.43,70.91 135.43,60.24 135.43,59.36 134.41,58.34 | 158.54,70.91 158.03,71.42 135.94,71.42 135.43,70.91 | 176.09,18.33 176.09,17.85 176.07,17.83 | 135.43,70.91 135.43,77.14 135.43,77.64
+24V
  Bottom 1.016: 134.76,18.72 LED3.A 134.89,18.72 U1.OUT+ JP30.1
+60
  Bottom 1.016: R69.1 73.83,35.76
  Bottom 1.27: R79.1 73.83,76.39 arc-45 73.91,76.57 74.59,77.26 76.78,77.26 arc-45 76.95,77.19 77.64,76.5 77.64,67.86 | 77.64,67.86 77.64,59.74 | 77.64,59.74 77.64,51.61 | 77.64,51.61 77.64,43.48 | 77.64,43.48 77.64,35.35 | 77.64,35.35 77.64,27.22 | 77.64,27.22 77.64,18.72 JP15.2 | R67.1 arc45 73.94,27.58 74.09,27.73 77.03,27.73 arc-45 77.21,27.66 77.64,27.22 | 73.83,35.76 73.88,35.76 arc45 74.06,35.83 74.09,35.86 77.03,35.86 arc-45 77.21,35.79 77.64,35.35 | R71.1 arc45 73.94,43.84 74.09,43.99 77.03,43.99 arc-45 77.21,43.91 77.64,43.48 | R73.1 arc45 73.94,51.97 74.09,52.12 77.03,52.12 arc-45 77.21,52.04 77.64,51.61 | R75.1 arc45 73.94,60.09 74.09,60.24 77.03,60.24 arc-45 77.21,60.17 77.64,59.74 | R77.1 arc45 73.94,68.22 74.09,68.37 77.03,68.37 arc-45 77.21,68.3 77.64,67.86
A-OUT
  Bottom 0.406: 123.24,65.83 IC3.1 | C17.2 R22.2
  Bottom 0.457: R12.2 123.24,65.83
  Bottom 0.61: R12.2 C17.2
  Bottom 1.016: R22.2 122.22,60.5 | 122.22,60.5 122.22,64.56 | 122.22,60.5 122.22,56.18 123.49,54.91 J1.1
D-OUT+5V
  Bottom 0.61: 130.79,42.46 130.79,42.91 130.86,42.97 131.49,42.34 | 130.79,42.46 130.79,41.64 130.22,41.07 IC8.3 | IC8.5 130.92,42.34 130.79,42.46
  Bottom 0.813: 124.25,52.37 J1.2 | 130.86,42.97 130.86,47.54 130.09,48.31 129.08,48.31 128.32,49.07 128.32,51.61 127.55,52.37 126.79,52.37
  Bottom 1.016: J1.2 126.54,52.37 126.79,52.62 R30.2 126.79,52.37 R32.1
GND  (via drill 0.8 pad 1.42, 1 pad 1.93, 1 pad 2.18, 3 pad 4)  (1 unrouted)
  Top 1.016: v187.75,70.15 v183.69,70.15 | v187.75,53.89 v183.69,53.89 | v187.75,37.64 v183.69,37.64 | v187.75,21.38 v183.69,21.38 | v166.16,63.04 v166.16,67.61 | v166.16,46.78 v166.16,51.35 | v166.16,30.53 v166.16,35.1 | v138.98,31.03 v134.92,31.03 | v154.99,33.07 v154.99,36.37 | v154.99,49.32 v154.99,52.62 | v153.97,65.58 v153.97,68.88 | v168.19,14.52 v168.19,19.35 | v139.24,14.27 v139.24,18.33 | v151.94,69.13 v151.94,73.71 | v138.98,47.04 v127.55,47.04 | v133.65,64.82 v137.21,64.82 | v133.27,77.01 v137.59,77.01 | v118.16,84.88 v118.16,80.82
  Bottom 0.406: 120.82,72.75 120.82,72.88 120.25,73.45 120.25,73.81 119.93,74.21 C7.2 118.66,74.21 118.26,75.65 | R11.2 126.35,64.62 125.14,65.83 IC2.4
  Bottom 0.61: R47.2 C55.1 | 151.14,32.81 C54.2 | IC9.4 143.81,28.75 143.3,29.26 142.85,29.26 C58.1 | C36.1 R33.2 154.92,48.63 | 151.14,49.07 C35.2 | IC6.4 143.81,45 143.3,45.51 142.85,45.51 C39.1 | R10.2 C10.1 | IC1.4 179.12,72.44 179.62,71.93 180.07,71.93 C8.1 | R31.2 C31.1 | IC5.4 179.12,56.18 179.62,55.67 180.07,55.67 C28.1 | C49.1 R46.2 168.01,36.3 | 171.79,35.86 C51.2 | IC7.4 179.12,39.92 179.62,39.42 180.07,39.42 C46.1 | R63.2 C68.1 | 171.79,19.6 C69.2 | IC10.4 179.12,23.67 179.62,23.16 180.07,23.16 C65.1 | R13.2 C18.1 | IC4.4 143.81,61.26 143.3,61.77 142.85,61.77 C21.1 | IC3.6 120.82,72.75 | IC2.4 125.14,69.52 125.01,69.64 | 118.66,74.98 118.26,75.65 117.9,76.25
  Bottom 0.813: 171.79,19.6 171.75,19.6 171.37,19.22 168.32,19.22 v168.19,19.35 168.01,19.54 R63.2 | C16.2 150.76,65.41 151.05,65.7 153.84,65.7 v153.97,65.58 154.6,65.58 154.92,65.26 R13.2 | 151.14,49.07 151.39,49.32 v154.99,49.32 154.99,47.74 R33.2 | C54.2 151.39,33.07 v154.99,33.07 154.92,33 R47.2
  Bottom 1.27: 161.59,35.1 162.1,34.59 164.13,34.59 | 157.53,57.2 159.94,59.61 JP20.1 | 157.02,40.18 160.19,43.35 JP24.1 | JP28.1 160.19,27.1 157.27,24.18
  Bottom 1.778: 36.24,27.26 D83.A D82.A D81.A D80.A D79.A 9.39,27.26 arc45 9.32,27.22 | 36.24,27.26 D84.A D85.A D86.A D87.A D88.A D89.A D90.A D91.A | D72.A D73.A D74.A D75.A D76.A D77.A D78.A | D72.A D71.A 35.99,35.38 | 35.99,35.38 D70.A D69.A D68.A D67.A D66.A 10.16,35.38 arc45 10.08,35.35 | D72.A 41.35,35.38 41.32,35.35 43.1,35.35 | 54.24,43.51 D62.A D63.A D64.A D65.A | 35.99,43.51 D58.A D59.A D60.A D61.A 54.24,43.51 | 35.99,43.51 D57.A D56.A D55.A D54.A D53.A 11.17,43.51 arc45 11.09,43.48 | 54.24,43.51 54.28,43.48 | D44.A D43.A D42.A D41.A D40.A 10.92,51.64 arc45 10.84,51.61 | D44.A 37.8,51.64 | 37.8,51.64 D45.A D46.A D47.A D48.A D49.A D50.A D51.A D52.A | 37.8,51.64 37.76,51.61 36.24,51.61 | 36.24,51.61 33.99,51.61 D44.A | 36.24,59.77 D31.A D30.A D29.A D28.A D27.A 9.39,59.77 arc45 9.32,59.74 | 36.24,59.77 D32.A D33.A D34.A D35.A D36.A D37.A D38.A D39.A | 35.99,67.9 D19.A D20.A D21.A D22.A D23.A D24.A D25.A D26.A | 35.99,67.9 D18.A D17.A D16.A D15.A D14.A 9.39,67.9 arc-45 9.21,67.97 | D13.A D12.A D11.A D10.A D9.A D8.A D7.A D6.A D5.A D4.A D3.A D2.A D1.A | JP11.1 arc-45 36.08,35.29 35.99,35.38 | JP13.1 36.24,27.26 | JP9.1 arc-45 36.08,43.42 35.99,43.51 | JP7.1 36.24,51.61 | JP3.1 arc-45 36.08,67.8 35.99,67.9 | JP5.1 36.24,59.77
  other vias: 186.1,85.9 112.82,86.03 185.97,12.62 112.69,12.75 11.86,85.9 11.98,12.62 85.01,12.75 84.88,86.03
  pour Bottom (isolate 0.406): 6.27,91.11 90.34,91.11 90.34,7.29 6.27,7.29
  pour Bottom (isolate 0.406): 191.31,91.11 107.23,91.11 107.49,7.29 191.31,7.29
N$1
  Bottom 0.61: R10.1 169.91,70.91 | 169.91,70.91 C10.2 | R9.2 170.48,70.78 | 170.48,70.78 170.03,70.78 169.91,70.91 | IC1.5 171.24,72.44 170.99,72.18 170.99,71.29 170.48,70.78
N$3
  Bottom 0.254: C5.1 C4.1
  Bottom 0.61: IC1.7 171.5,74.98 170.99,75.48 169.72,75.48 | 169.72,75.48 168.96,75.48 | 168.96,75.48 168.16,75.48 C4.1 | R6.1 169.97,75.74 169.72,75.48 | C2.1 169.59,77.9 168.96,77.26 168.96,75.48
N$4
  Bottom 1.27: U2.IN+ 137.21,80.06 134.41,82.85 115.11,82.85 112.57,80.31 112.57,49.26 115.11,46.72 J2.1
N$5
  Bottom 1.016: R79.2 73.83,73.45 | 73.83,73.45 R78.1 | C77.1 73.96,73.33 arc-90 73.83,73.45
N$6
  Bottom 0.61: R7.1 C8.2 180.07,73.71 IC1.3 176.32,73.71 175.81,73.2 175.81,71.11 R8.2
N$7
  Bottom 0.61: C2.2 R2.2
N$8
  Bottom 0.61: IC1.6 170.23,73.71 | 170.23,73.71 170.16,73.71 | 170.16,73.71 R6.2 170.03,73.9 170.23,73.71 | 170.16,73.71 168.13,73.71 C5.2 C4.2 167.94,73.71 C9.2
N$9
  Bottom 0.61: C3.2 R3.2 179.82,75.93 178.86,74.98 IC1.2 176.32,74.98 175.81,75.48 175.81,77.83 R2.1
N$10
  Bottom 0.61: C3.1 R3.1 177.91,77.83 177.59,77.52 | D92.A 178.35,79.8 177.59,79.04 177.59,77.52 | 177.59,77.52 177.59,76.31 IC1.1
N$12  (via drill 1 pad 2.18)
  Top 1.016: v137.97,60.37 v127.3,60.37
  Bottom 0.61: IC2.2 127.68,65.7 128.32,65.07 128.25,65 R11.1 R18.1 128.25,61.83
  Bottom 0.813: 128.25,61.83 128.25,61.32 v127.3,60.37
  Bottom 1.016: 136.95,41.7 136.95,25.45 | D96.C 137.39,42.14 136.95,41.7 | D98.C 137.39,25.88 136.95,25.45 | 185.72,31.54 185.72,17.57 184.45,16.3 138.22,16.3 136.95,17.57 136.95,25.45 | 185.72,31.54 185.72,47.8 | 185.72,47.8 185.72,63.04 | D97.C 185.21,31.03 185.72,31.54 | D95.C 185.21,47.29 185.72,47.8 | D93.C 185.21,63.55 185.72,63.04 | 136.95,41.7 136.95,53.39 | D94.C 137.46,53.89 136.95,53.39 | 136.95,53.39 136.95,56.94 137.97,57.96 v137.97,60.37 | D92.C 184.7,79.8 185.72,78.79 185.72,63.04
N$13
  Bottom 1.016: R77.2 73.83,65.32 | 73.83,65.32 R76.1 | C76.1 73.96,65.2 arc-90 73.83,65.32
N$14
  Bottom 1.016: R75.2 73.83,56.94 | 73.83,56.94 R74.1 | C75.1 73.96,57.07 arc90 73.83,56.94
N$15
  Bottom 1.016: R73.2 73.83,48.81 | 73.83,48.81 R72.1 | C74.1 73.96,48.94 arc90 73.83,48.81
N$16
  Bottom 1.016: R71.2 73.83,40.69 | 73.83,40.69 R70.1 | C73.1 73.96,40.81 arc90 73.83,40.69
N$17
  Bottom 1.016: R69.2 73.83,32.81 | 73.83,32.81 R68.1 | C72.1 73.96,32.69 arc-90 73.83,32.81
N$18
  Bottom 1.016: R67.2 73.83,24.68 | 73.83,24.68 R66.1 | C71.1 73.96,24.56 arc-90 73.83,24.68
N$23
  Bottom 0.61: IC2.1 128.95,66.72 129.59,66.09 129.59,57.96 128.82,57.2 127.55,57.2 126.79,56.43 R30.1
N$24
  Bottom 0.406: 124.25,68.12 124.25,65.07 124.19,65.07 R12.1
  Bottom 0.61: 124.25,64.63 R12.1 C17.1 R18.2 | IC3.2 122.09,68.25 122.47,68.63 123.74,68.63 124.25,68.12
N$25
  Bottom 0.61: IC2.3 126.41,67.99 127.05,68.63 133.58,68.63 C13.1
  Bottom 1.016: R65.S C13.1
N$26
  Bottom 1.016: R65.E 131.11,77.26 130.09,76.25 R4.2
N$27
  Bottom 1.016: R65.A 131.11,63.61 R15.1
N$28
  Bottom 0.61: IC5.6 170.23,57.45 | 170.23,57.45 170.16,57.45 | 170.16,57.45 R24.2 170.03,57.64 170.23,57.45 | 170.16,57.45 168.13,57.45 C26.2 C25.2 167.94,57.45 C29.2
N$29
  Bottom 1.016: R64.E 118.28,78.91 119.49,77.7 119.49,76.5 R5.1
N$30
  Bottom 1.016: R64.A 114.6,63.61 R14.2
N$31
  Bottom 0.61: IC3.3 120.82,68.25 120.44,68.63 117.9,68.63 117.14,69.39 117.14,71.17 | R64.S 117.14,71.17 | C11.2 117.14,71.17
N$32
  Bottom 1.016: LED1.C R1.1
N$33
  Bottom 0.61: R31.1 169.91,54.66 | 169.91,54.66 C31.2 | R29.2 170.48,54.53 | 170.48,54.53 170.03,54.53 169.91,54.66 | IC5.5 171.24,56.18 170.99,55.93 170.99,55.04 170.48,54.53
N$34
  Bottom 1.016: LED3.C 134.69,22.37 133.9,23.16 133.9,24.24 | R56.1 133.9,24.24 | 133.9,24.24 R57.1
N$35
  Bottom 0.254: C25.1 C26.1
  Bottom 0.61: IC5.7 171.5,58.72 170.99,59.23 169.72,59.23 | 169.72,59.23 168.96,59.23 | 168.96,59.23 168.16,59.23 C25.1 | R24.1 169.97,59.48 169.72,59.23 | C19.1 169.59,61.64 168.96,61.01 168.96,59.23
N$36
  Bottom 0.61: C19.2 R19.2
N$37
  Bottom 0.61: C22.2 R21.2 179.82,59.67 178.86,58.72 IC5.2 176.32,58.72 175.81,59.23 175.81,61.58 R19.1
N$38
  Bottom 0.254: IC5.1 177.59,60.05
  Bottom 0.61: C22.1 R21.1 177.91,61.58 177.59,61.26 | 177.59,60.05 177.59,61.26 | 177.59,61.26 177.59,62.53 178.61,63.55 D93.A
N$39
  Bottom 0.61: R26.1 C28.2 180.07,57.45 IC5.3 176.32,57.45 175.81,56.94 175.81,54.85 R28.2
N$40
  Bottom 0.61: IC6.6 152.7,43.73 | 152.7,43.73 152.76,43.73 | 152.76,43.73 R39.2 152.89,43.54 152.7,43.73 | 152.76,43.73 154.79,43.73 | 154.79,43.73 C42.2 C41.2 154.99,43.73 | C38.2 154.79,43.73
N$41
  Bottom 0.61: R33.1 153.02,46.53 | 153.02,46.53 C36.2 | R34.2 152.45,46.66 | 152.45,46.66 152.89,46.66 153.02,46.53 | IC6.5 151.68,45 151.94,45.26 151.94,46.15 152.45,46.66
N$42
  Bottom 0.61: IC7.6 170.23,41.19 | 170.23,41.19 170.16,41.19 | 170.16,41.19 R40.2 170.03,41.39 170.23,41.19 | 170.16,41.19 168.13,41.19 C44.2 C43.2 167.94,41.19 C47.2
N$43
  Bottom 0.61: R46.1 169.91,38.4 | 169.91,38.4 C49.2 | R45.2 170.48,38.27 | 170.48,38.27 170.03,38.27 169.91,38.4 | IC7.5 171.24,39.92 170.99,39.67 170.99,38.78 170.48,38.27
N$44
  Bottom 0.254: C43.1 C44.1
  Bottom 0.61: IC7.7 171.5,42.46 170.99,42.97 169.72,42.97 | 169.72,42.97 168.96,42.97 | 168.96,42.97 168.16,42.97 C43.1 | R40.1 169.97,43.23 169.72,42.97 | C37.1 169.59,45.39 168.96,44.75 168.96,42.97
N$45
  Bottom 0.61: C37.2 R36.2
N$46
  Bottom 0.61: C40.2 R38.2 179.82,43.42 178.86,42.46 IC7.2 176.32,42.46 175.81,42.97 175.81,45.32 R36.1
N$47
  Bottom 0.61: C40.1 R38.1 177.91,45.32 177.59,45 | D95.A 178.35,47.29 177.59,46.53 177.59,45 | 177.59,45 177.59,43.79 IC7.1
N$48
  Bottom 0.61: R42.1 C46.2 180.07,41.19 IC7.3 176.32,41.19 175.81,40.69 175.81,38.59 R44.2
N$49
  Bottom 0.254: C42.1 C41.1
  Bottom 0.61: IC6.7 151.43,42.46 151.94,41.96 153.21,41.96 | 153.21,41.96 153.97,41.96 | 153.97,41.96 154.77,41.96 C41.1 | R39.1 152.95,41.7 153.21,41.96 | C48.1 153.33,39.54 153.97,40.18 153.97,41.96
N$50
  Bottom 0.61: C48.2 R43.2
N$51
  Bottom 0.61: IC10.6 170.23,24.94 | 170.23,24.94 170.16,24.94 | 170.16,24.94 R55.2 170.03,25.13 170.23,24.94 | 170.16,24.94 168.13,24.94 C63.2 C62.2 167.94,24.94 C66.2
N$52
  Bottom 0.61: R63.1 169.91,22.14 | 169.91,22.14 C68.2 | R62.2 170.48,22.02 | 170.48,22.02 170.03,22.02 169.91,22.14 | IC10.5 171.24,23.67 170.99,23.41 170.99,22.52 170.48,22.02
N$53
  Bottom 0.254: C62.1 C63.1
  Bottom 0.61: IC10.7 171.5,26.21 170.99,26.72 169.72,26.72 | 169.72,26.72 168.96,26.72 | 168.96,26.72 168.16,26.72 C62.1 | R55.1 169.97,26.97 169.72,26.72 | C56.1 169.59,29.13 168.96,28.49 168.96,26.72
N$54
  Bottom 0.61: C56.2 R50.2
N$55
  Bottom 0.61: C59.2 R53.2 179.82,27.16 178.86,26.21 IC10.2 176.32,26.21 175.81,26.72 175.81,29.06 R50.1
N$56
  Bottom 0.61: C59.1 R53.1 177.97,29.06 177.65,28.75 | IC10.1 177.65,28.75 | 177.65,28.75 177.65,30.33 178.35,31.03 D97.A
N$57
  Bottom 0.61: R59.1 C65.2 180.07,24.94 IC10.3 176.32,24.94 175.81,24.43 175.81,22.34 R61.2
N$58
  Bottom 0.61: C45.2 R41.2 143.11,41.51 144.06,42.46 IC6.2 146.6,42.46 147.11,41.96 147.11,39.61 R43.1
N$59
  Bottom 0.61: IC6.1 145.27,40.88 144,39.61 R41.1 C45.1 139.1,39.61 D96.A
N$60
  Bottom 0.61: IC4.6 152.7,59.99 | 152.7,59.99 152.76,59.99 | 152.76,59.99 R23.2 152.89,59.8 152.7,59.99 | 152.76,59.99 154.79,59.99 | 154.79,59.99 C24.2 C23.2 154.99,59.99 | C20.2 154.79,59.99
N$61
  Bottom 0.61: R13.1 153.02,62.78 | 153.02,62.78 C18.2 | R16.2 152.45,62.91 | 152.45,62.91 152.89,62.91 153.02,62.78 | IC4.5 151.68,61.26 151.94,61.51 151.94,62.4 152.45,62.91
N$62
  Bottom 0.254: C23.1 C24.1
  Bottom 0.61: IC4.7 151.43,58.72 151.94,58.21 153.21,58.21 | 153.21,58.21 153.97,58.21 | 153.97,58.21 154.77,58.21 C23.1 | R23.1 152.95,57.96 153.21,58.21 | C30.1 153.33,55.8 153.97,56.43 153.97,58.21
N$63
  Bottom 0.61: C30.2 R27.2
N$64
  Bottom 0.61: C27.2 R25.2 143.11,57.77 144.06,58.72 IC4.2 146.6,58.72 147.11,58.21 147.11,55.86 R27.1
N$65
  Bottom 0.61: C27.1 141.97,55.86 | IC4.1 145.27,57.14 144,55.86 R25.1 142.29,55.86 | 142.29,55.86 141.97,55.86 | 141.97,55.86 141.78,55.67 | D94.A 141.78,53.97 141.78,55.36 142.29,55.86
N$66
  Bottom 0.61: R20.1 C21.2 142.85,59.99 IC4.3 146.6,59.99 147.11,60.5 147.11,62.59 R17.2
N$67
  Bottom 0.61: R37.1 C39.2 142.85,43.73 IC6.3 146.6,43.73 147.11,44.24 147.11,46.34 R35.2
N$69
  Bottom 0.61: IC9.6 152.7,27.48 | 152.7,27.48 152.76,27.48 | 152.76,27.48 R54.2 152.89,27.29 152.7,27.48 | 152.76,27.48 154.79,27.48 | 154.79,27.48 C61.2 C60.2 154.99,27.48 | C57.2 154.79,27.48
N$70
  Bottom 0.61: R47.1 153.02,30.27 | 153.02,30.27 C55.2 | R48.2 152.45,30.4 | 152.45,30.4 152.89,30.4 153.02,30.27 | IC9.5 151.68,28.75 151.94,29 151.94,29.89 152.45,30.4
N$71
  Bottom 0.254: C60.1 C61.1
  Bottom 0.61: IC9.7 151.43,26.21 151.94,25.7 153.21,25.7 | 153.21,25.7 153.97,25.7 | 153.97,25.7 154.77,25.7 C60.1 | R54.1 152.95,25.45 153.21,25.7 | C67.1 153.33,23.29 153.97,23.92 153.97,25.7
N$72
  Bottom 0.61: C67.2 R60.2
N$73
  Bottom 0.61: C64.2 R58.2 143.11,25.25 144.06,26.21 IC9.2 146.6,26.21 147.11,25.7 147.11,23.35 R60.1
N$74
  Bottom 0.61: IC9.1 145.27,24.62 144,23.35 R58.1 C64.1 139.1,23.35 D98.A
N$75
  Bottom 0.61: R52.1 C58.2 142.85,27.48 IC9.3 146.6,27.48 147.11,27.99 147.11,30.08 R49.2
N$78
  Bottom 0.61: IC8.1 128.26,38.71 | 128.26,39.16 IC8.2 | 128.26,38.71 128.32,38.65 | 128.26,38.71 IC8.2 | 127.74,39.1 127.74,39.29 IC8.2
  Bottom 0.813: SP1.+ 118.66,39.16 127.68,39.16 127.74,39.1
N$79
  Bottom 0.406: IC8.6 IC8.7
  Bottom 0.61: 133.4,40.43 133.4,39.86 IC8.7 133.46,40.88 133.4,40.94 133.4,40.43 | 133.4,40.43 131.62,40.43 130.35,39.16 130.35,30.53 128.57,28.75 R51.2
OUT1
  Bottom 1.016: R74.2 72.73,54.09 arc-45 72.55,54.16 72.31,54.4 D39.C
  Bottom 1.778: D27.C D28.C D29.C D30.C D31.C 36.24,54.4 | 36.24,54.4 D32.C D33.C D34.C D35.C D36.C D37.C D38.C D39.C | JP6.1 36.24,54.4
OUT3
  Bottom 1.016: R66.2 72.73,21.58 arc-45 72.55,21.65 72.31,21.89 D91.C
  Bottom 1.778: D91.C D90.C D89.C D88.C D87.C D86.C D85.C D84.C 36.24,21.89 | 36.24,21.89 D83.C D82.C D81.C D80.C D79.C | JP14.1 36.24,21.89
OUT4
  Bottom 1.016: R78.2 72.73,70.34 arc-45 72.55,70.42 72.31,70.66 D13.C
  Bottom 1.778: 35.99,70.66 D6.C D7.C D8.C D9.C D10.C D11.C D12.C D13.C | 35.99,70.66 D5.C D4.C D3.C D2.C D1.C | JP2.1 36.24,71.02 arc-45 36.17,70.84 35.99,70.66
OUT5
  Bottom 1.016: R76.2 72.73,62.22 arc-45 72.55,62.29 72.31,62.53 D26.C
  Bottom 1.778: D26.C D25.C D24.C D23.C D22.C D21.C D20.C D19.C 36.5,62.53 | 36.5,62.53 D18.C D17.C D16.C D15.C D14.C | JP4.1 36.24,62.89 arc45 36.31,62.71 36.5,62.53
OUT9
  Bottom 1.016: R72.2 72.73,45.96 arc-45 72.55,46.03 72.31,46.27 D52.C
  Bottom 1.778: D40.C D41.C D42.C D43.C D44.C 35.73,46.27 | 35.73,46.27 D45.C D46.C D47.C D48.C D49.C D50.C D51.C D52.C | JP8.1 36.22,46.66 arc45 36.04,46.58 35.73,46.27
OUT10
  Bottom 1.016: C9.1 161.72,70.91 JP17.1
OUT12
  Bottom 1.016: JP19.1 157.14,62.91 C20.1
OUT13
  Bottom 1.016: C66.1 161.72,22.14 JP29.1
OUT14
  Bottom 1.016: C29.1 161.72,54.65 JP21.1
OUT15
  Bottom 1.016: 161.46,46.53 JP23.1 161.47,46.53 C38.1
OUT16
  Bottom 1.016: C47.1 161.72,38.4 JP25.1
OUT17
  Bottom 1.016: JP27.1 157.14,30.4 C57.1
OUT21
  Bottom 1.016: R70.2 72.73,37.83 arc-45 72.55,37.91 72.31,38.15 D65.C
  Bottom 1.778: D65.C D64.C D63.C D62.C D61.C D60.C D59.C D58.C 36.24,38.15 | 36.24,38.15 D57.C D56.C D55.C D54.C D53.C | JP10.1 36.24,38.15
OUT22
  Bottom 1.016: R68.2 72.73,29.7 arc-45 72.55,29.78 72.31,30.02 D78.C
  Bottom 1.778: D66.C D67.C D68.C D69.C D70.C | D70.C D71.C D72.C D73.C D74.C D75.C D76.C D77.C D78.C | D70.C 35.75,30.02 arc45 35.93,30.09 JP12.1
S$1
  Bottom 0.61: IC3.7 122.09,70.53 121.71,70.15 119.68,70.15 119.43,70.4 119.43,71.86 IC3.5
S$2
  Bottom 0.61: R51.1 LED2.A
S$3  (via drill 3 pad 4)
  other vias: 131.36,53
S$4  (via drill 3 pad 4)
  other vias: 116.12,23.29

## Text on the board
Bottom: SEMICONDUCTOR RADIATION DETECTOR / & GAMMA ANALYZER V1 PROT. BPW34 MATRIX | SEMICONDUCTOR RADIATION DETECTOR / & GAMMA ANALYZER / V1 PROT. BPW34 MATRIX | Design: Marcin Wachowiak, Poland | Design: Marcin Wachowiak, Poland
tPlace: D1-D91 / BPW34
tNames: SEMICONDUCTOR RADIATION DETECTOR / & GAMMA ANALYZER / V1 PROT. BPW34 MATRIX | Design: Marcin Wachowiak, Poland | Design: Marcin Wachowiak, Poland

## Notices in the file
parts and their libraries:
diy-modules: Released under the Creative Commons Attribution 4.0 International License: http://creativecommons.org/licenses/by/4.0
